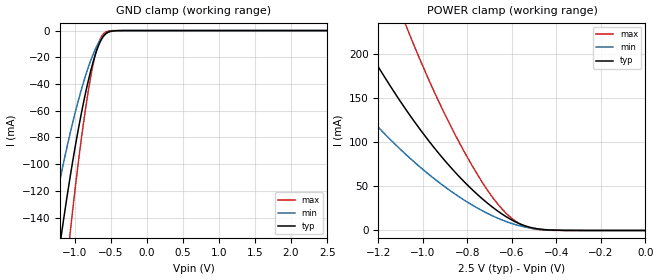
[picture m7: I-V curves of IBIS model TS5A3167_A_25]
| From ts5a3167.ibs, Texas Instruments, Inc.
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[Model]   TS5A3167_A_25
Model_type  Terminator
| variable   typ   min   max
C_comp   18.78pF   17.11pF   20.33pF
| C_tri-state   18.78pF   17.11pF   20.33pF
[Temperature Range]   40   100   -40
| Ambient temperature   25   85   -40
[Voltage range]   2.5   2.3   2.7
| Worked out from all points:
|   GND clamp passes 1 mA (typ) near -0.53 V on its own axis
|   POWER clamp passes 1 mA (typ) near -0.46 V on its own axis
[GND Clamp]
| TS5A3167_A_25
|   Voltage   I(typ)   I(min)   I(max)
-2.5V     -831.8mA   -595.1mA   -1.147A
-1.34V    -215.6mA   -150mA     -306.8mA
-1.19V    -155.5mA   -108.5mA   -219.3mA
-1.165V   -146.1mA   -102mA     -205.6mA
-1.06V    -109.1mA   -76.54mA   -150.8mA
-900mV    -60.3mA    -43.07mA   -78.53mA
-785mV    -32.05mA   -23.62mA   -37.15mA
-680mV    -12.92mA   -10.32mA   -11.51mA
-625mV    -6.385mA   -5.542mA   -4.338mA
-575mV    -2.755mA   -2.678mA   -1.33mA
-395mV    -33.36uA   -60.36uA   -3.018uA
2.5V      746.8pA    2.254uA    48.2pA
[POWER Clamp]
| TS5A3167_A_25
|   Voltage   I(typ)   I(min)   I(max)
-2.5V     969.5mA    652.7mA    1.529A
-1.565V   359.7mA    230.6mA    603.2mA
-1.3V     228.8mA    144.9mA    388.3mA
-1.075V   136.8mA    85.92mA    231.9mA
-1.055V   129.5mA    81.31mA    219.4mA
-905mV    80.35mA    50.24mA    133.8mA
-800mV    51.62mA    32.19mA    82.95mA
-690mV    27mA       16.93mA    38.61mA
-600mV    11.84mA    7.867mA    13.57mA
-540mV    5.17mA     3.876mA    4.537mA
-470mV    1.358mA    1.283mA    755uA
-31.15fV  746.8pA    6.23nA     61.57pA
